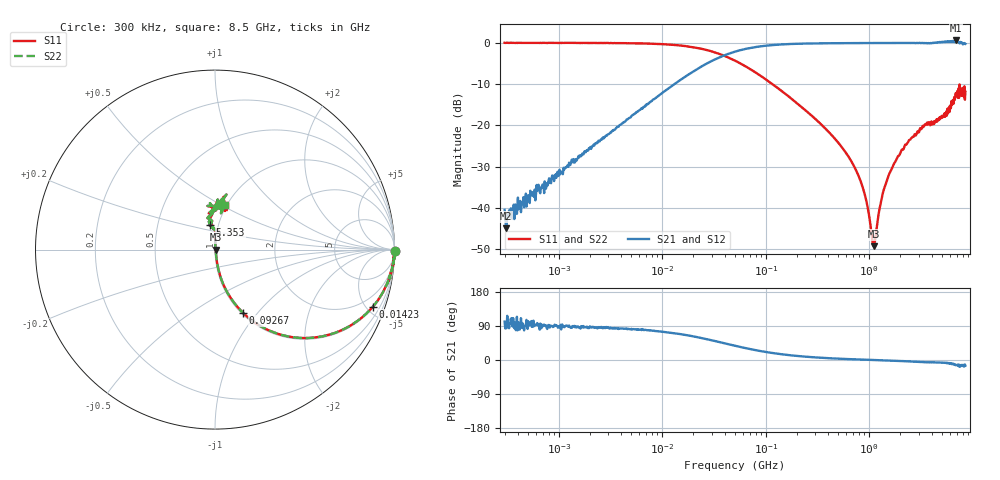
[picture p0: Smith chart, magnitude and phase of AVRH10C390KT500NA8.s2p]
! S-Parameter Data Generated by TDK Corporation
! Copyright(C) 2023 TDK Corporation.
! All Rights Reserved.
! TDK P/N: AVRH10C390KT500NA8 (Varistor)
! Property: V1mA=39V
! Size(LxWxT): 1x0.5x0.5mm
! Model Type: s2p (Touchstone File Format Version 1.0)
! Frequency: DC=Yes Start=0.3MHz Stop=8500MHz 802points Log-sweep
! Model Generated on Oct. 12, 2023
! Port Assignments:
!  1 ---N--- 2
! Applicable Conditions:
!  Temperature = 25 degC
!  DC Bias Voltage = 0 V
!  Small Signal Operation
! Terms and conditions regarding TDK Simulation Models
! (1)This simulation model is being provided solely for informational purposes. Please refer to the specifications of the products in terms of detailed characteristics of such products.
! (2)In no event shall TDK Corporation of any of its subsidiaries be liable for any loss or damage arising, directly or indirectly,
!  From any information contained in this simulation model, including, but not limited to loss or damages arising from any inaccuracies, omissions or errors in connection with such information.
! (3)Any and all copyrights on this simulation model are owned by TDK Corporation.
!  Duplication or redistribution of this simulation model without prior written permission from TDK Corporation is prohibited.
! (4)This simulation model is subject to any modification or change without any prior notice.
! (5)Neither TDK Corporation nor any of its subsidiaries shall make any warranty, express or implied,
!  Including but not limited to the correctness, implied warranties of merchantability and fitness for a particular purpose with respect to this simulation models.
! (6)The use of this simulation model shall be deemed to have consented to the terms and conditions hereof.
# Hz S MA R 50
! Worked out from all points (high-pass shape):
!   801 points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, 300 kHz to 8.5 GHz, reference 50 ohm
!   highest |S21| = 0.59 dB at 6.906 GHz (marker M1); lowest = -44.9 dB at 309 kHz (marker M2)
!   |S21| within 3 dB of the highest: 46.47 MHz to end of sweep
!   lowest |S11| = -49.2 dB at 1.106 GHz (marker M3), VSWR 1.01, Z = 50.3 + j0.0284 ohm
!   |S11| at or under -10 dB: 116.4 MHz to end of sweep
!   |S22| runs from -49.2 to 0.0 dB; largest |S21 - S12| = 0
!   S11 on the Smith chart (normalised r, x): 300 kHz: open; 14.23 MHz: 1.09, -5.49; 92.67 MHz: 1.02, -0.85; 5.353 GHz: 0.91, +0.26; 8.5 GHz: 0.98, +0.53
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300000  1.002 -0.5  0.009495 101.2  0.009495 101.2  1.002 -0.5
309002  1.001 -0.3  0.005702 96.6  0.005702 96.6  1.001 -0.3
1667340  0.9985 -2.5  0.04379 86.8  0.04379 86.8  0.9985 -2.5
9160260  0.9696 -13.1  0.227 75.8  0.227 75.8  0.9696 -13.1
1.42299e7  0.9347 -19.9  0.3404 69.2  0.3404 69.2  0.9347 -19.9
2.98011e7  0.7916 -36.9  0.5999 52.3  0.5999 52.3  0.7916 -36.9
5.11488e7  0.6048 -51.9  0.7869 37.2  0.7869 37.2  0.6048 -51.9
9.26665e7  0.3868 -66.0  0.9138 22.8  0.9138 22.8  0.3868 -66.0
2.80466e8  0.1301 -79.5  0.9848 7.5  0.9848 7.5  0.1301 -79.5
5.10608e8  0.06035 -81.0  0.9924 3.4  0.9924 3.4  0.06035 -81.0
7.33302e8  0.03002 -78.5  0.9945 1.7  0.9945 1.7  0.03002 -78.5
8.82652e8  0.01639 -73.0  0.9953 0.9  0.9953 0.9  0.01639 -73.0
1.06509e9  0.004346 -33.1  0.9964 0.1  0.9964 0.1  0.004346 -33.1
1.10624e9  0.00345 4.7  0.9966 -0.0  0.9966 -0.0  0.00345 4.7
1.14739e9  0.004349 41.4  0.9967 -0.2  0.9967 -0.2  0.004349 41.4
1.31613e9  0.01292 79.4  0.9977 -0.7  0.9977 -0.7  0.01292 79.4
1.54289e9  0.02497 85.9  0.9985 -1.4  0.9985 -1.4  0.02497 85.9
2.49786e9  0.06747 85.7  0.9973 -3.9  0.9973 -3.9  0.06747 85.7
3.44114e9  0.1027 83.1  0.9929 -5.9  0.9929 -5.9  0.1027 83.1
5.35322e9  0.1408 101.5  1.037 -7.6  1.037 -7.6  0.1408 101.5
6.90594e9  0.2469 99.8  1.07 -13.1  1.07 -13.1  0.2469 99.8
8.5e9  0.2565 76.9  0.9742 -14.9  0.9742 -14.9  0.2565 76.9
